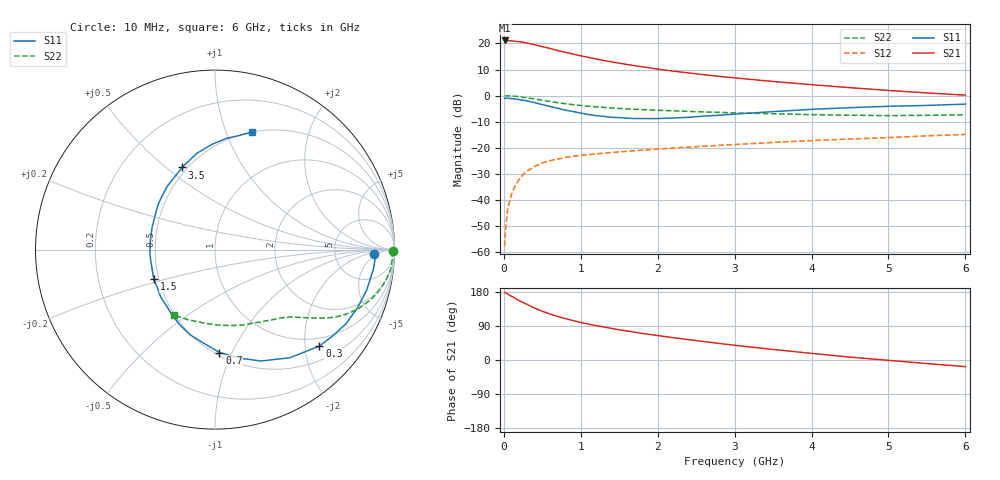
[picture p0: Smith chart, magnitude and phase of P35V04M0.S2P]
! SIEMENS Small Signal Semiconductors
! BFP181
! Si NPN RF Bipolar Junction Transistor in SOT143
! VCE = 5 V  IC = 4 mA
! Common Emitter S-Parameters:  March  1996
# GHz  S  MA  R  50
!  f  S11  S21  S12  S22
! GHz  MAG  ANG  MAG  ANG  MAG  ANG  MAG  ANG
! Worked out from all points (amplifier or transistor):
!   36 points, 10 MHz to 6 GHz, reference 50 ohm
!   highest |S21| = 21.1 dB at 10 MHz (marker M1)
!   |S21| within 3 dB of that: start of sweep to 592.7 MHz
!   unconditionally stable (mu >= 1): 1.937 GHz to end of sweep
!   at 250 MHz: K = 0.19, MSG = 25.4 dB, |S12| = -30.3 dB
!   at 1.4 GHz: K = 0.83, MSG = 17.4 dB, |S12| = -21.8 dB
!   at 6 GHz: K = 1.06, MAG = 6.0 dB, |S12| = -14.9 dB
!   S11 on the Smith chart (normalised r, x): 10 MHz: 16, -4; 300 MHz: 0.80, -2.32; 700 MHz: 0.52, -0.90; 1.5 GHz: 0.47, -0.18; 3.5 GHz: 0.47, +0.57; 6 GHz: 0.50, +1.23
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0.01  0.885 -1.6  11.4 178.6  0.0013 90.4  0.9926 -0.6
0.02  0.8945 -2.9  11.37 177.9  0.0026 83.6  0.9866 -1.2
0.05  0.8892 -7.1  11.32 174.0  0.0068 86.6  0.989 -3.3
0.1  0.8747 -14.9  11.16 168.3  0.0129 81.8  0.984 -6.6
0.2  0.8384 -29.6  10.81 156.9  0.0249 74.4  0.9518 -12.7
0.25  0.8138 -36.1  10.48 151.5  0.0305 70.2  0.9303 -15.6
0.3  0.7922 -42.7  10.16 147.0  0.0355 66.9  0.9084 -18.1
0.4  0.7328 -55.3  9.439 137.1  0.0438 61.1  0.8621 -22.6
0.5  0.6715 -67.6  8.683 128.5  0.051 55.6  0.8151 -26.2
0.6  0.6181 -77.7  8.024 121.4  0.0566 51.7  0.7708 -29.1
0.7  0.5739 -87.5  7.28 115.1  0.061 48.6  0.7318 -31.4
0.9  0.4952 -106.1  6.26 104.0  0.0689 43.6  0.6712 -34.6
1.1  0.4333 -124.0  5.413 94.6  0.074 40.5  0.6248 -37.3
1.3  0.4008 -139.3  4.706 86.9  0.0787 38.4  0.5922 -39.5
1.5  0.379 -154.1  4.188 79.7  0.0832 37.0  0.5664 -41.4
1.8  0.3636 -175.8  3.557 70.1  0.0899 35.6  0.539 -44.7
2.2  0.3715 160.8  2.945 58.9  0.0985 33.7  0.5108 -49.5
2.8  0.4207 134.3  2.338 43.6  0.1115 31.1  0.4775 -57.8
3.5  0.4932 111.8  1.863 27.8  0.1265 27.9  0.4492 -69.2
4.5  0.5868 91.6  1.419 7.6  0.1471 22.4  0.42 -89.2
5.5  0.6484 78.3  1.126 -9.4  0.1691 17.4  0.4186 -110.7
6  0.6862 72.6  1.02 -17.5  0.1805 14.1  0.4294 -121.8
